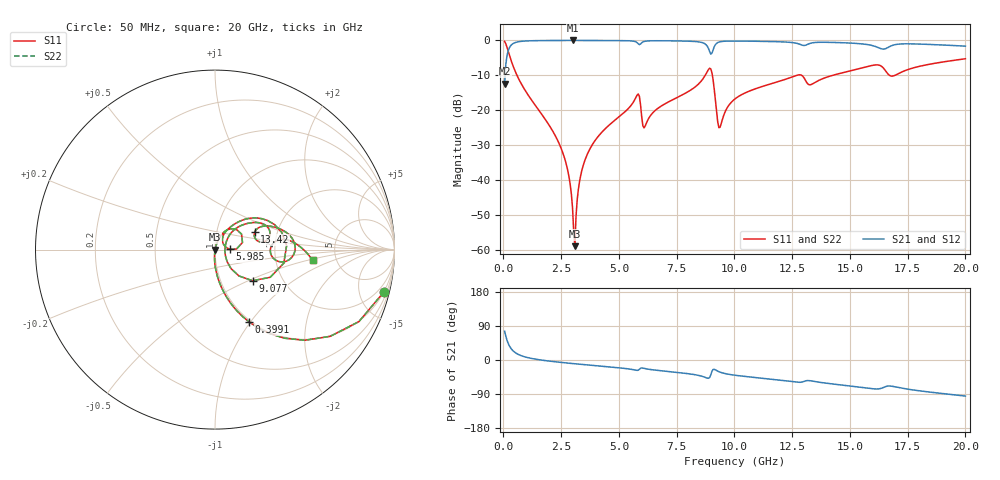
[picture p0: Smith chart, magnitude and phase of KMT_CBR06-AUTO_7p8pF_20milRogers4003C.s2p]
! Data measured by Modelithics Inc. support@modelithics.com 813-866-6335
! KEMET CBR06-AUTO 7.8pF, Pad Width= 0.851mm, Pad Length= 0.64mm, Pad Gap= 0.62mm, 20mil Rogers 4003C substrate Data, January 2022
# hz S ma R 50
! 2 Port Network Data from SP1.SP block
! freq  magS11  angS11  magS21  angS21  magS12  angS12  magS22  angS22
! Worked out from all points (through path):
!   401 points, 50 MHz to 20 GHz, reference 50 ohm
!   highest |S21| = -0.01 dB at 2.993 GHz (marker M1); lowest = -12.4 dB at 50 MHz (marker M2)
!   group delay of S21, straight-line fit = 14.4 ps
!   lowest |S11| = -58.9 dB at 3.092 GHz (marker M3), VSWR 1.00, Z = 50.1 + j0.0522 ohm
!   |S11| at or under -10 dB: 586.3 MHz to 8.735 GHz (8.149 GHz wide, 175 % of centre); 9.045 GHz to 12.7 GHz (3.653 GHz wide, 33.6 % of centre); 12.91 GHz to 14.25 GHz (1.342 GHz wide, 9.88 % of centre)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
!   |S22| runs from -58.9 to -0.3 dB; largest |S21 - S12| = 0
!   S11 on the Smith chart (normalised r, x): 50 MHz: 0.98, -8.01; 399.1 MHz: 0.98, -0.99; 5.985 GHz: 1.18, +0.00; 9.077 GHz: 1.41, -0.53; 13.42 GHz: 1.53, +0.32; 20 GHz: 3.31, -0.55
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5e7  0.9708 -14.0  0.2397 76.0  0.2397 76.0  0.9708 -14.0
3.99125e8  0.4464 -64.7  0.8942 25.2  0.8942 25.2  0.4464 -64.7
2.493875e9  0.02868 -94.7  0.9987 -6.4  0.9987 -6.4  0.02868 -94.7
2.793125e9  0.01327 -94.5  0.999 -8.2  0.999 -8.2  0.01327 -94.5
2.992625e9  0.003926 -86.4  0.999 -9.4  0.999 -9.4  0.003926 -86.4
3.092375e9  0.001131 27.4  0.999 -10.0  0.999 -10.0  0.001131 27.4
3.391625e9  0.01364 74.3  0.9988 -11.7  0.9988 -11.7  0.01364 74.3
3.990125e9  0.0378 73.4  0.9981 -15.0  0.9981 -15.0  0.0378 73.4
5.73575e9  0.1528 49.4  0.9525 -26.9  0.9525 -26.9  0.1528 49.4
5.985125e9  0.08108 1.0  0.9241 -20.9  0.9241 -20.9  0.08108 1.0
6.13475e9  0.0593 43.4  0.9743 -22.7  0.9743 -22.7  0.0593 43.4
6.73325e9  0.1094 59.8  0.9891 -27.8  0.9891 -27.8  0.1094 59.8
8.678375e9  0.2948 36.7  0.9114 -44.6  0.9114 -44.6  0.2948 36.7
9.077375e9  0.2716 -39.7  0.7347 -24.9  0.7347 -24.9  0.2716 -39.7
9.376625e9  0.05698 10.1  0.9567 -32.0  0.9567 -32.0  0.05698 10.1
1.0025e10  0.1453 46.1  0.9796 -40.2  0.9796 -40.2  0.1453 46.1
1.271825e10  0.3178 23.7  0.9053 -58.5  0.9053 -58.5  0.3178 23.7
1.336662e10  0.2371 22.5  0.923 -55.5  0.923 -55.5  0.2371 22.5
1.34165e10  0.2422 23.9  0.9287 -56.1  0.9287 -56.1  0.2422 23.9
1.605988e10  0.444 4.6  0.8281 -76.3  0.8281 -76.3  0.444 4.6
1.670825e10  0.317 -6.3  0.8118 -68.6  0.8118 -68.6  0.317 -6.3
2e10  0.5464 -6.1  0.828 -95.2  0.828 -95.2  0.5464 -6.1
